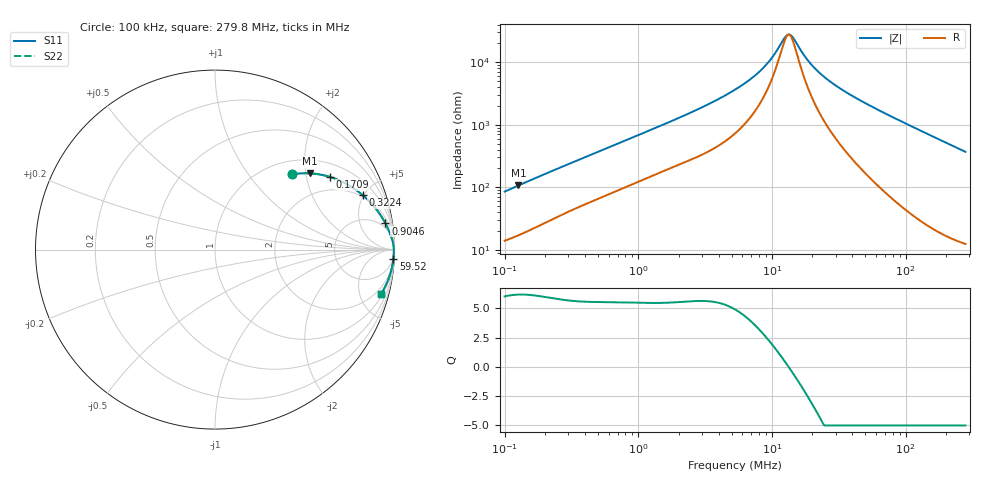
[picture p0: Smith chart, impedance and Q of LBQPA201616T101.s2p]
! LBQPA201616T101  S-PARAMETER MODEL  ( General Type )
! Model Generated by TAIYO YUDEN Corporation (http://www.ty-top.com)
! Version 1.0
! TAIYO YUDEN Control No. 191025NI43SB-FBB
! Copyright(c) 2019 TAIYO YUDEN CO.,LTD. All Rights Reserved.
! Product Description (link to TY-COMPAS)
! https://ds.yuden.co.jp/TYCOMPAS/or/detail?pn=LBQPA201616T101K&u=M
! Products Name : Inductors
! Characteristics :
!  Inductance : 100 uH , SRF(min) : 8.0 MHz , DC Resistance(max) : 10.4 Ohm
!  Rated Current : Saturation :110 mA , Temp Rise : 95 mA (20 degC)
!  Case Size : 2.0 x 1.6 / 0.079 x 0.063 [mm/inch] , Thickness : 1.6 / 0.063 [mm/inch]
!  (Conditions: Temperature = 25 degC , DC Bias Current/Voltage = 0A / 0V)
! External Node Assignments :
!  1  o---GGG---o  2
! GND o---------o GND
! Frequency Range : 0.1MHz  -  279.750408MHz  [ 402 STEP ]
# MHz S RI R 50
! Freq[MHz].  S11 Real  S11 Imag  S21 Real  S21 Imag  S12 Real  S12 Imag  S22 Real  S22 Imag
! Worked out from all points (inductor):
!   401 points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, 100 kHz to 279.8 MHz, reference 50 ohm
!   read as one part in series: L = 132 uH near 104 kHz
!   highest Q = 6.19 at 126.9 kHz (marker M1), where L = 132 uH
!   self-resonance near 13.18 MHz
!   S11 on the Smith chart (normalised r, x): 100 kHz: 1.28, +1.67; 170.9 kHz: 1.45, +2.78; 322.4 kHz: 1.87, +4.91; 904.6 kHz: 3, +12; 59.52 MHz: 3, -36; 279.8 MHz: 1.25, -7.36
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0.1  0.43 0.4191  0.57 -0.4191  0.57 -0.4191  0.43 0.4191
0.126883  0.5269 0.425  0.4731 -0.425  0.4731 -0.425  0.5269 0.425
0.170867  0.6424 0.4043  0.3576 -0.4043  0.3576 -0.4043  0.6424 0.4043
0.322403  0.8225 0.3037  0.1775 -0.3037  0.1775 -0.3037  0.8225 0.3037
0.377863  0.8529 0.2759  0.1471 -0.2759  0.1471 -0.2759  0.8529 0.2759
0.904646  0.9497 0.1458  0.0503 -0.1458  0.0503 -0.1458  0.9497 0.1458
1.427803  0.9709 0.0999  0.0291 -0.0999  0.0291 -0.0999  0.9709 0.0999
3.03467  0.9884 0.0502  0.0116 -0.0502  0.0116 -0.0502  0.9884 0.0502
5.289144  0.9938 0.0267  0.00617 -0.0267  0.00617 -0.0267  0.9938 0.0267
6.982683  0.9951 0.0176  0.00485 -0.0176  0.00485 -0.0176  0.9951 0.0176
8.685774  0.9958 0.0113  0.00421 -0.0113  0.00421 -0.0113  0.9958 0.0113
10.17991  0.9961 0.00699  0.0039 -0.00699  0.0039 -0.00699  0.9961 0.00699
12.41404  0.9964 0.00183  0.00365 -0.00183  0.00365 -0.00183  0.9964 0.00183
13.17541  0.9964 0.000301  0.0036 -0.000301  0.0036 -0.000301  0.9964 0.000301
14.26368  0.9965 -0.00174  0.00354 0.00174  0.00354 0.00174  0.9965 -0.00174
17.39406  0.9965 -0.00692  0.00349 0.00692  0.00349 0.00692  0.9965 -0.00692
19.9857  0.9965 -0.0107  0.00351 0.0107  0.00351 0.0107  0.9965 -0.0107
30.31621  0.9961 -0.0236  0.00389 0.0236  0.00389 0.0236  0.9961 -0.0236
59.51829  0.9935 -0.0545  0.00646 0.0545  0.00646 0.0545  0.9935 -0.0545
75.51853  0.9914 -0.0703  0.00862 0.0703  0.00862 0.0703  0.9914 -0.0703
148.2617  0.9754 -0.1389  0.0246 0.1389  0.0246 0.1389  0.9754 -0.1389
279.7504  0.924 -0.2487  0.076 0.2487  0.076 0.2487  0.924 -0.2487
